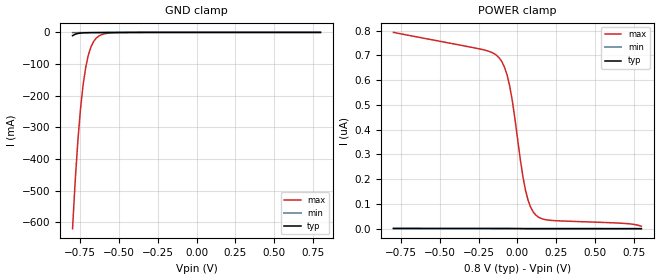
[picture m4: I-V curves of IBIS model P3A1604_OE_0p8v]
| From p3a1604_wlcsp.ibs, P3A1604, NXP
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[Model] P3A1604_OE_0p8v
Model_type Input
Polarity   Non-Inverting
Enable   Active-High
Vinl =  0.365V
Vinh =  0.411V
C_comp   2.027pF   1.667pF   2.300pF
[Model Spec]
Vinh   0.411V   0.331V   0.499V
Vinl   0.365V   0.283V   0.443V
[Temperature Range]   27.000   -40.000   125
[Voltage Range]   0.800V   0.720V   0.880V
[POWER Clamp Reference]   0.800V   0.720V   0.880V
[GND Clamp Reference]   0.0V   0.0V   0.0V
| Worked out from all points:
|   GND clamp passes 1 mA (typ) near -0.70 V on its own axis
[GND_clamp]
|Voltage   I(typ)   I(min)   I(max)
-800mV    -10.35mA   -806.7uA   -619.6mA
-783mV    -5.842mA   -738.2uA   -469.8mA
-766mV    -3.455mA   -685.3uA   -344.1mA
-749mV    -2.187mA   -639.3uA   -243.2mA
-732mV    -1.506mA   -596.5uA   -166.1mA
-715mV    -1.131mA   -555.2uA   -110.1mA
-698mV    -914.4uA   -515uA     -71.33mA
-681mV    -781uA     -475.4uA   -45.45mA
-664mV    -690.9uA   -436.5uA   -28.69mA
-630mV    -568.2uA   -360.7uA   -11.39mA
-494mV    -241.4uA   -99.63uA   -655.5uA
800mV     0A         0A         0A
[POWER_clamp]
|Voltage   I(typ)   I(min)   I(max)
-800mV    1.043nA    183.5pA    793.3nA
-220mV    860.7pA    101.6pA    723.1nA
-118mV    822.7pA    87.08pA    690.8nA
-84mV     793.7pA    81.42pA    654nA
-50mV     723.3pA    72.36pA    577.4nA
-33mV     657.3pA    64.27pA    517.9nA
35mV      265pA      13.74pA    212.8nA
52mV      205.5pA    8.208pA    156.4nA
86mV      146.8pA    4.063pA    85.91nA
120mV     127.2pA    2.968pA    54.19nA
205mV     114.9pA    1.943pA    34.2nA
800mV     0A         0A         9.793nA
